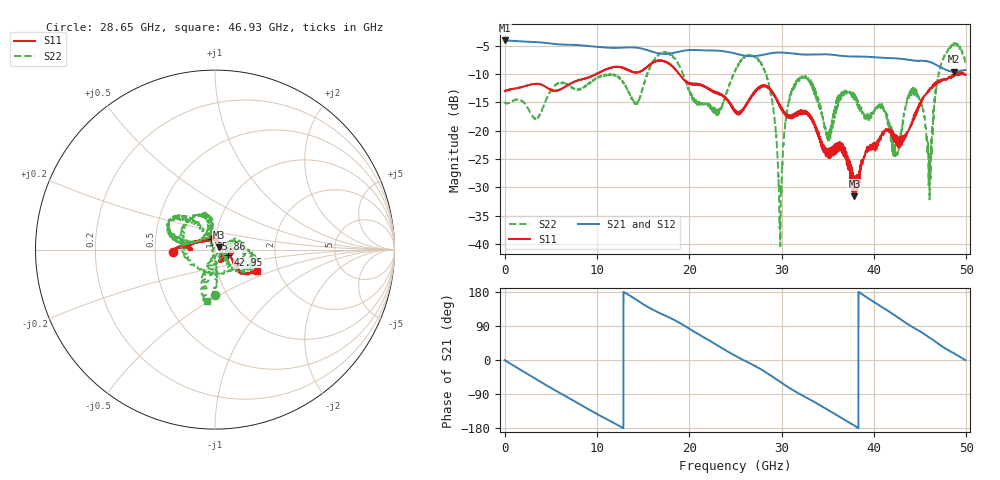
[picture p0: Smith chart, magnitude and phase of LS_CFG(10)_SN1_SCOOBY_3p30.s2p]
!Keysight Technologies,N5245B,MY58422026,A.13.80.08
!Date: Thursday, March 19, 2020 23:29:47
!Correction: S11(Full 2 Port(1,2))
!S21(Full 2 Port(1,2))
!S12(Full 2 Port(1,2))
!S22(Full 2 Port(1,2))
!S2P File: Measurements: S11, S21, S12, S22:
# Hz S DB R 50.0
!freq dBS11 angS11 dBS21 angS21 dBS12 angS12 dBS22 angS22
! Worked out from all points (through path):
!   4991 points, 10 MHz to 49.91 GHz, reference 50 ohm
!   highest |S21| = -4.07 dB at 20 MHz (marker M1); lowest = -9.6 dB at 48.67 GHz (marker M2)
!   group delay of S21, straight-line fit = 39.7 ps
!   lowest |S11| = -31.6 dB at 37.89 GHz (marker M3), VSWR 1.05, Z = 52.4 + j1.24 ohm
!   |S11| at or under -10 dB: start of sweep to 9.919 GHz; 18.89 GHz to 48.66 GHz (29.77 GHz wide, 88.1 % of centre); 48.67085 GHz to 48.75742 GHz (86.57 MHz wide, 0.178 % of centre)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
!   |S22| runs from -40.4 to -4.5 dB; largest |S21 - S12| = 0.0059
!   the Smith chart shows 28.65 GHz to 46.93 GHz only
!   S11 on the Smith chart (normalised r, x): 28.65 GHz: 0.62, -0.02; 35.86 GHz: 0.95, +0.11; 42.95 GHz: 1.15, -0.07; 46.93 GHz: 1.56, -0.40
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1e7  -13.00 -1.0  -4.08 -0.3  -4.06 -0.3  -14.90 0.2
2e7  -12.98 -0.5  -4.07 -0.4  -4.06 -0.4  -15.02 -0.5
4.3e9  -12.09 -53.4  -4.48 -63.3  -4.47 -63.3  -15.41 -81.6
8.33e9  -11.01 -78.9  -4.94 -119.4  -4.94 -119.4  -12.58 -85.6
1.427e10  -9.69 -125.7  -5.34 159.0  -5.33 159.0  -15.13 -133.8
1.665e10  -7.64 -135.7  -6.33 125.5  -6.33 125.5  -6.67 -163.7
2.299e10  -13.47 -164.9  -5.86 39.7  -5.86 39.8  -17.04 -164.4
2.496e10  -16.51 -161.9  -6.36 11.4  -6.35 11.5  -9.53 -173.2
2.865e10  -12.58 -177.0  -6.39 -37.8  -6.39 -37.7  -12.02 -90.5
2.986e10  -15.97 174.4  -6.20 -58.0  -6.20 -57.8  -40.41 153.6
3.093e10  -17.66 -179.1  -6.31 -75.0  -6.31 -74.8  -13.85 130.6
3.328e10  -17.69 160.5  -6.56 -107.2  -6.56 -106.9  -11.88 164.3
3.504e10  -24.52 114.3  -6.54 -132.0  -6.49 -131.6  -21.62 128.1
3.586e10  -24.14 111.0  -6.65 -143.8  -6.59 -143.5  -17.26 104.4
3.789e10  -31.61 26.9  -6.91 -173.0  -6.85 -173.1  -14.08 156.3
4.16e10  -19.88 -5.0  -7.19 128.5  -7.21 128.3  -19.01 27.9
4.295e10  -22.14 -22.6  -7.32 106.6  -7.35 106.5  -20.70 -48.3
4.445e10  -16.78 -34.4  -7.62 83.2  -7.64 83.3  -12.91 -16.7
4.603e10  -12.68 -36.5  -7.85 59.1  -7.87 59.2  -32.16 -39.7
4.693e10  -11.55 -26.6  -8.54 43.8  -8.55 43.8  -10.73 -99.1
4.867e10  -10.00 -49.2  -9.60 17.6  -9.62 17.7  -4.59 -58.5
4.991e10  -10.16 -45.3  -9.29 -0.5  -9.31 -0.7  -7.83 -25.2
